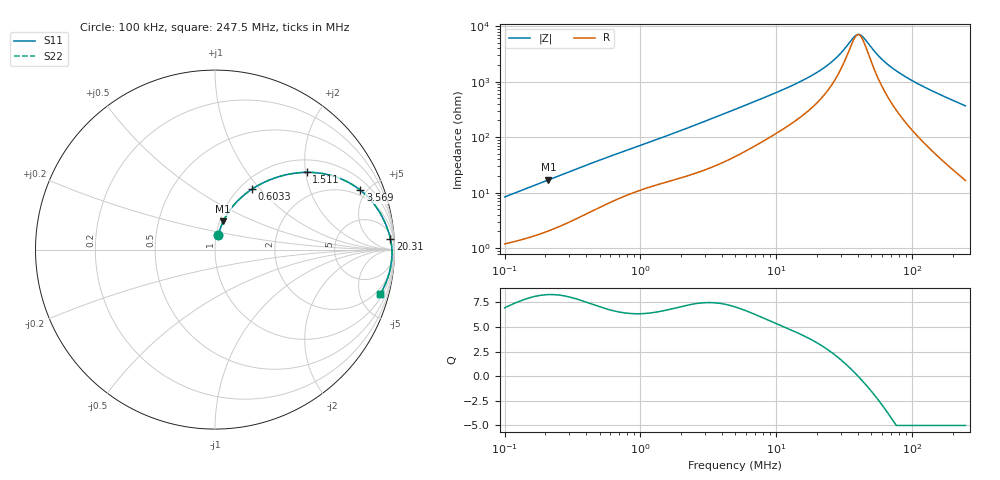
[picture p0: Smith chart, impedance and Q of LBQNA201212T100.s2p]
! LBQNA201212T100  S-PARAMETER MODEL  ( General Type )
! Model Generated by TAIYO YUDEN Corporation (http://www.ty-top.com)
! Version 1.0
! TAIYO YUDEN Control No. 191025NI43SB-FBB
! Copyright(c) 2019 TAIYO YUDEN CO.,LTD. All Rights Reserved.
! Product Description (link to TY-COMPAS)
! https://ds.yuden.co.jp/TYCOMPAS/or/detail?pn=LBQNA201212T100K&u=M
! Products Name : Inductors
! Characteristics :
!  Inductance : 10 uH , SRF(min) : 32 MHz , DC Resistance(max) : 0.91 Ohm
!  Rated Current : Saturation :190 mA , Temp Rise : 300 mA (20 degC)
!  Case Size : 2.0 x 1.25 / 0.079 x 0.049 [mm/inch] , Thickness : 1.25 / 0.049 [mm/inch]
!  (Conditions: Temperature = 25 degC , DC Bias Current/Voltage = 0A / 0V)
! External Node Assignments :
!  1  o---GGG---o  2
! GND o---------o GND
! Frequency Range : 0.1MHz  -  247.502633MHz  [ 402 STEP ]
# MHz S RI R 50
! Freq[MHz].  S11 Real  S11 Imag  S21 Real  S21 Imag  S12 Real  S12 Imag  S22 Real  S22 Imag
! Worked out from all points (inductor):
!   401 points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, 100 kHz to 247.5 MHz, reference 50 ohm
!   read as one part in series: L = 13.1 uH near 104 kHz
!   highest Q = 8.28 at 210.1 kHz (marker M1), where L = 12.8 uH
!   self-resonance near 40.12 MHz
!   S11 on the Smith chart (normalised r, x): 100 kHz: 1.02, +0.17; 603.3 kHz: 1.13, +0.90; 1.511 MHz: 1.30, +2.03; 3.569 MHz: 1.61, +4.55; 20.31 MHz: 10, +29; 247.5 MHz: 1.33, -7.33
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0.1  0.0184 0.0803  0.9816 -0.0803  0.9816 -0.0803  0.0184 0.0803
0.210083  0.0462 0.1581  0.9538 -0.1581  0.9538 -0.1581  0.0462 0.1581
0.37019  0.1058 0.2492  0.8942 -0.2492  0.8942 -0.2492  0.1058 0.2492
0.603286  0.2047 0.3358  0.7953 -0.3358  0.7953 -0.3358  0.2047 0.3358
1.370406  0.4729 0.4288  0.5271 -0.4288  0.5271 -0.4288  0.4729 0.4288
1.511016  0.5109 0.4305  0.4891 -0.4305  0.4891 -0.4305  0.5109 0.4305
2.233305  0.6624 0.4087  0.3376 -0.4087  0.3376 -0.4087  0.6624 0.4087
3.569133  0.81 0.3309  0.19 -0.3309  0.19 -0.3309  0.81 0.3309
4.974964  0.8786 0.2632  0.1214 -0.2632  0.1214 -0.2632  0.8786 0.2632
11.08235  0.956 0.129  0.044 -0.129  0.044 -0.129  0.956 0.129
18.41681  0.975 0.0708  0.025 -0.0708  0.025 -0.0708  0.975 0.0708
20.30646  0.9774 0.0611  0.0226 -0.0611  0.0226 -0.0611  0.9774 0.0611
27.22034  0.9827 0.0339  0.0173 -0.0339  0.0173 -0.0339  0.9827 0.0339
30.60534  0.9841 0.0235  0.0159 -0.0235  0.0159 -0.0235  0.9841 0.0235
37.20803  0.9857 0.00654  0.0143 -0.00654  0.0143 -0.00654  0.9857 0.00654
40.23208  0.9861 -0.000243  0.0139 0.000243  0.0139 0.000243  0.9861 -0.000243
43.50191  0.9863 -0.00706  0.0137 0.00706  0.0137 0.00706  0.9863 -0.00706
56.07892  0.9862 -0.0299  0.0138 0.0299  0.0138 0.0299  0.9862 -0.0299
68.1772  0.9851 -0.0488  0.0149 0.0488  0.0149 0.0488  0.9851 -0.0488
86.18795  0.9822 -0.0738  0.0178 0.0738  0.0178 0.0738  0.9822 -0.0738
113.2979  0.9761 -0.1078  0.0239 0.1078  0.0239 0.1078  0.9761 -0.1078
247.5026  0.9211 -0.2478  0.0789 0.2478  0.0789 0.2478  0.9211 -0.2478
